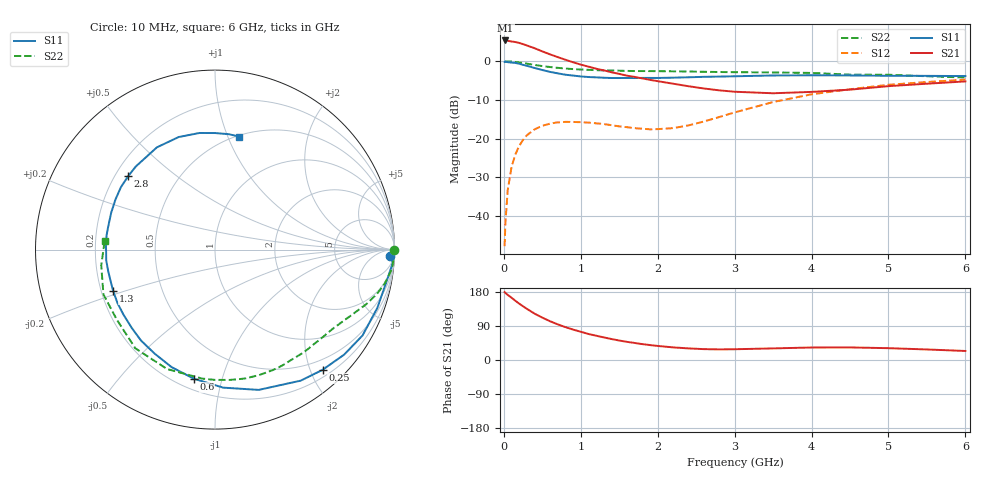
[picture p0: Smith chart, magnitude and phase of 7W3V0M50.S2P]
! Infineon Technologies  Discrete & RF Semiconductors
! BFS17W
! Si NPN RF Bipolar Junction Transistor in SOT323
! VCE = 3 V  IC = 0.5 mA
! Common Emitter S-Parameters:  August  1999
# GHz  S  MA  R  50
!  f  S11  S21  S12  S22
! GHz  MAG  ANG  MAG  ANG  MAG  ANG  MAG  ANG
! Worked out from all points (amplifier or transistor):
!   36 points, 10 MHz to 6 GHz, reference 50 ohm
!   highest |S21| = 5.4 dB at 20 MHz (marker M1)
!   |S21| within 3 dB of that: start of sweep to 523.1 MHz
!   unconditionally stable (mu >= 1): 1.197 GHz to end of sweep
!   at 250 MHz: K = 0.22, MSG = 12.4 dB, |S12| = -20.3 dB
!   at 1.4 GHz: K = 1.17, MAG = 4.3 dB, |S12| = -16.5 dB
!   at 6 GHz: K = 1.10, MAG = -2.2 dB, |S12| = -4.8 dB
!   S11 on the Smith chart (normalised r, x): 10 MHz: 26, -41; 250 MHz: 0.32, -2.20; 600 MHz: 0.27, -0.81; 1.3 GHz: 0.25, -0.18; 2.8 GHz: 0.25, +0.35; 6 GHz: 0.51, +1.10
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0.01  0.9778 -2.0  1.831 179.2  0.0041 87.3  0.9999 -0.1
0.02  0.9934 -4.2  1.855 176.9  0.0081 89.9  0.9914 -1.2
0.05  0.9733 -10.1  1.835 171.9  0.0215 84.7  0.996 -3.0
0.1  0.961 -19.8  1.799 164.4  0.0433 77.8  0.9922 -5.9
0.15  0.9511 -30.2  1.77 156.2  0.0626 71.6  0.9775 -8.8
0.25  0.8988 -48.2  1.663 141.6  0.0966 60.9  0.9471 -13.7
0.3  0.8725 -56.8  1.597 134.9  0.1109 56.5  0.9311 -15.8
0.4  0.8187 -72.7  1.472 122.3  0.1321 48.2  0.8963 -19.8
0.5  0.7704 -86.6  1.34 111.9  0.1468 41.2  0.8663 -22.9
0.6  0.7289 -99.3  1.228 102.3  0.1566 35.9  0.8424 -25.8
0.8  0.6701 -120.1  1.046 86.8  0.1648 28.1  0.8052 -31.2
1.1  0.6255 -144.7  0.852 68.7  0.1614 21.7  0.7742 -38.8
1.3  0.6124 -157.9  0.763 59.6  0.1547 20.4  0.7612 -44.3
1.6  0.6091 -174.4  0.651 47.9  0.1408 22.8  0.7503 -52.6
2.2  0.6138 160.5  0.513 33.3  0.137 43.3  0.7412 -70.7
2.8  0.6337 139.8  0.421 28.0  0.1905 60.3  0.726 -89.9
3.5  0.6552 119.6  0.386 30.6  0.2974 61.6  0.717 -111.9
4  0.659 107.9  0.402 33.0  0.3743 55.9  0.7067 -128.9
4.5  0.6555 97.6  0.43 33.2  0.4353 49.0  0.672 -144.5
5  0.6494 90.0  0.477 31.2  0.4965 42.2  0.6699 -158.1
5.5  0.6476 83.2  0.513 27.8  0.5394 35.5  0.6399 -172.1
6  0.6437 77.8  0.549 23.8  0.5786 29.2  0.6168 175.8
